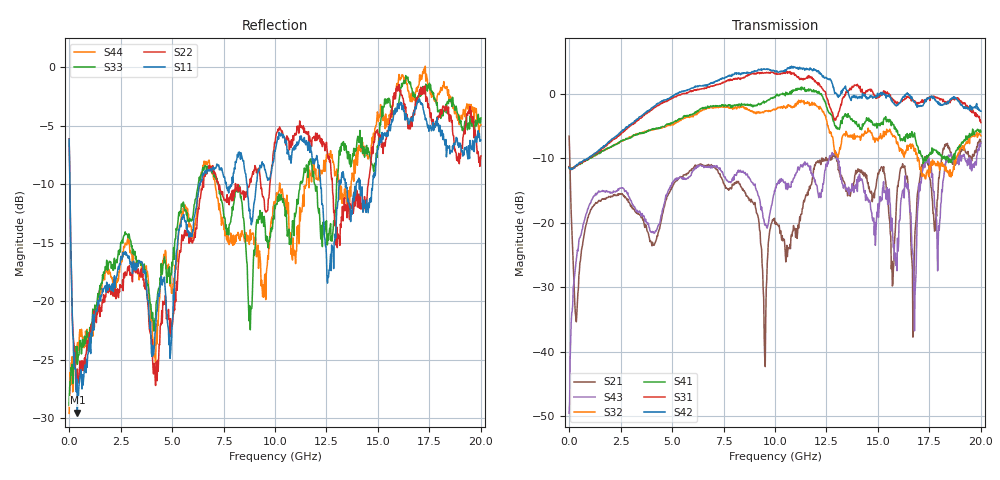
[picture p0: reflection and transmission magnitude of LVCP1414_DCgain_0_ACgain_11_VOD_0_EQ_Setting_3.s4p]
!Agilent Technologies,N5230A,MY46400459,A.07.50.48
!Agilent N5230A: A.07.50.48
!Date: Tuesday, April 17, 2012 18:38:02
!Correction: S11(Full 4 Port(1,2,3,4))
!S12(Full 4 Port(1,2,3,4))
!S13(Full 4 Port(1,2,3,4))
!S14(Full 4 Port(1,2,3,4))
!S21(Full 4 Port(1,2,3,4))
!S22(Full 4 Port(1,2,3,4))
!S23(Full 4 Port(1,2,3,4))
!S24(Full 4 Port(1,2,3,4))
!S31(Full 4 Port(1,2,3,4))
!S32(Full 4 Port(1,2,3,4))
!S33(Full 4 Port(1,2,3,4))
!S34(Full 4 Port(1,2,3,4))
!S41(Full 4 Port(1,2,3,4))
!S42(Full 4 Port(1,2,3,4))
!S43(Full 4 Port(1,2,3,4))
!S44(Full 4 Port(1,2,3,4))
!S4P File: Measurements: <S11,S12,S13,S14>,
!<S21,S22,S23,S24>,
!<S31,S32,S33,S34>,
!<S41,S42,S43,S44>:
# Hz S  dB  R 50
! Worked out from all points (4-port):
!   801 points, 300 kHz to 20 GHz, reference 50 ohm
!   strongest paths, dB at 300 kHz, 5 GHz, 10 GHz, 15 GHz, 20 GHz:
!     S42: -11.4, -0.4, 3.4, 0.0, -2.7
!     S31: -11.3, -0.7, 3.1, -0.6, -4.5
!     S41: -11.3, -4.5, -0.6, -4.6, -5.9
!     S32: -11.3, -4.8, -2.5, -7.3, -6.5
!     S43: -49.5, -13.8, -15.1, -17.1, -7.6
!     S21: -6.6, -14.5, -20.2, -12.3, -7.5
!   lowest |S11| = -29.5 dB at 400.3 MHz (marker M1), VSWR 1.07, Z = 53.1 + j1.52 ohm
!   |S11| at or under -10 dB: 37.49 MHz to 6.322 GHz (6.284 GHz wide, 198 % of centre); 12.21 GHz to 13.11 GHz (899.5 MHz wide, 7.1 % of centre); 14.13 GHz to 14.75 GHz (614.3 MHz wide, 4.25 % of centre)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
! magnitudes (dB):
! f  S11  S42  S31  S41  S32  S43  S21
! 300 kHz  -6.1  -11.4  -11.3  -11.3  -11.3  -49.5  -6.6
! 400.3 MHz  -29.5  -11.0  -11.0  -11.1  -11.1  -24.2  -32.4
! 6.275 GHz  -10.7  1.1  0.7  -2.6  -2.9  -11.1  -11.2
! 9.5 GHz  -8.8  3.8  3.2  -1.3  -2.7  -20.3  -40.8
! 12.73 GHz  -17.4  2.1  -2.5  -3.3  -6.0  -9.7  -9.8
! 16.8 GHz  -3.5  -1.2  -1.1  -6.7  -8.5  -31.2  -21.4
! 20 GHz  -6.2  -2.7  -4.5  -5.9  -6.5  -7.6  -7.5
